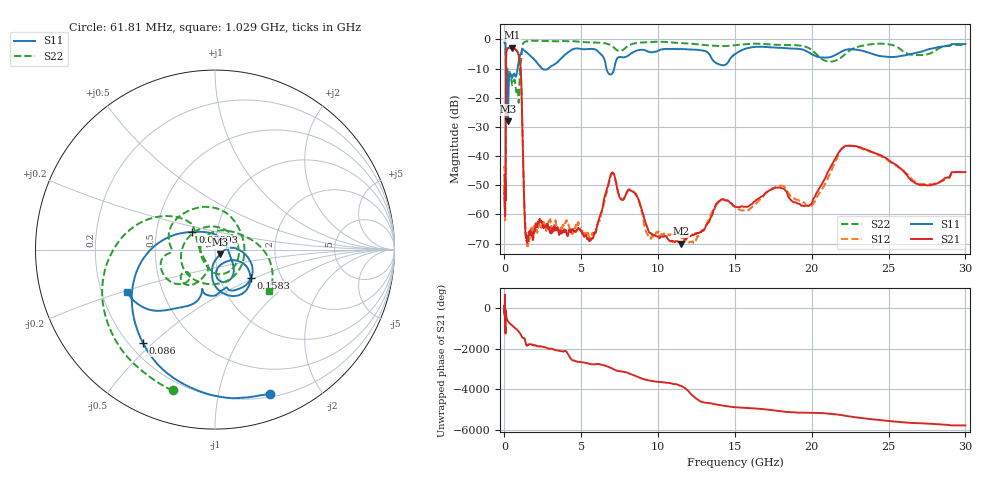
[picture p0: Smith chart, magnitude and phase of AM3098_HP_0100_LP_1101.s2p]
! Date/Time: Thu, Feb 28, 2019 8:35 AM
! Network Analyzer: Agilent Technologies E8364B Rev: A.07.50.67
! Sweep from 0.010 to 30.000 GHz, 1601 Points, Sweep Type: LOG
! Power Supply: 5.023 V, 0.002 A
# Hz S DB R 50
!freq MagS11 AngS11 MagS21 AngS21 MagS12 AngS12 MagS22 AngS22
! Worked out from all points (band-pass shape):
!   1601 points, 10 MHz to 30 GHz, reference 50 ohm
!   highest |S21| = -2.78 dB at 490.6 MHz (marker M1); lowest = -70.0 dB at 11.48 GHz (marker M2)
!   |S21| within 3 dB of the highest: 112.4 MHz to 944.6 MHz (832.2 MHz wide, 157 % of centre)
!   lowest |S11| = -28.1 dB at 235.1 MHz (marker M3), VSWR 1.08, Z = 52.9 - j2.81 ohm
!   |S11| at or under -10 dB: 95.96 MHz to 849.6 MHz (753.6 MHz wide, 159 % of centre); 2.457 GHz to 2.838 GHz (380.7 MHz wide, 14.4 % of centre); 6.639 GHz to 7.14 GHz (500.5 MHz wide, 7.26 % of centre)
!   |S22| runs from -22.2 to -0.4 dB; largest |S21 - S12| = 0.01
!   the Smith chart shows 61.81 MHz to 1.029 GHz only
!   S11 on the Smith chart (normalised r, x): 61.81 MHz: 0.23, -1.43; 86 MHz: 0.25, -0.46; 98.93 MHz: 0.76, +0.15; 158.3 MHz: 1.40, -0.47; 1.029 GHz: 0.31, -0.21
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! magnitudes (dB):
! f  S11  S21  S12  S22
! 10 MHz  -0.3  -46.3  -44.3  -0.6
! 38.04 MHz  -0.5  -60.1  -59.6  -1.0
! 61.81 MHz  -1.3  -53.2  -49.5  -1.7
! 76.65 MHz  -2.1  -54.8  -53.7  -2.6
! 86 MHz  -3.7  -38.5  -37.9  -4.0
! 98.93 MHz  -15.9  -12.9  -12.8  -20.1
! 144.7 MHz  -16.8  -3.6  -3.6  -13.5
! 158.3 MHz  -11.9  -3.5  -3.4  -11.2
! 235.1 MHz  -28.1  -2.9  -2.9  -12.1
! 490.6 MHz  -13.2  -2.8  -2.8  -15.5
! 550.5 MHz  -12.4  -3.0  -3.0  -15.0
! 926.3 MHz  -7.8  -5.4  -5.3  -21.7
! 1.029 GHz  -5.3  -8.7  -8.6  -8.4
! 1.369 GHz  -4.1  -66.3  -64.1  -0.7
! 2.084 GHz  -7.7  -64.0  -65.5  -0.5
! 5.584 GHz  -3.2  -68.9  -68.2  -1.0
! 6.924 GHz  -12.0  -46.2  -46.9  -2.0
! 7.926 GHz  -5.9  -53.0  -52.8  -2.7
! 11.48 GHz  -3.3  -70.0  -67.6  -1.2
! 19.8 GHz  -4.5  -57.1  -57.1  -2.9
! 22.56 GHz  -3.4  -36.5  -36.5  -3.5
! 30 GHz  -1.6  -45.5  -45.4  -1.9
